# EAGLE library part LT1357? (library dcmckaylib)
High-speed (25MHz), high slew rate (600V/us) High bias current, 8nV/Hz^(0.5) voltage noise
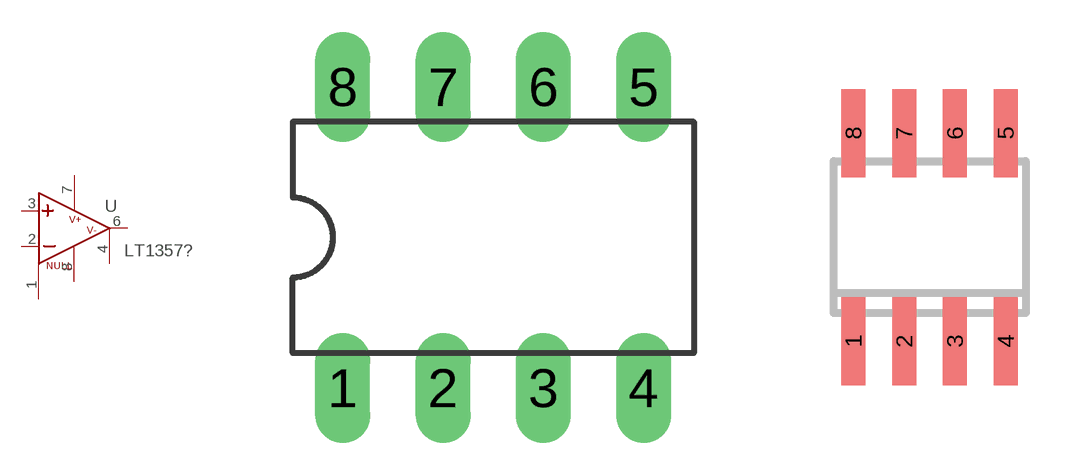
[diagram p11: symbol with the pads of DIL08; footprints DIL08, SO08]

Designator prefix U

## LT1357CN8  [DIL08]
1  NULL1
2  IN-  in
3  IN+  in
4  V-  pwr
6  OUT  out
7  V+  pwr
8  NULL2

## LT1357C38  [SO08]
Pads as for DIL08

## Footprint DIL08 (pad centres in mm)
Dual In Line Package
drill 0.889 long: 1 -3.81,-3.81; 2 -1.27,-3.81; 3 1.27,-3.81; 4 3.81,-3.81; 5 3.81,3.81; 6 1.27,3.81; 7 -1.27,3.81; 8 -3.81,3.81

## Footprint SO08 (pad centres in mm)
Small Outline Package 8 NS Package M08A
smd 0.6 x 2.2: 1 -1.905,-2.6; 2 -0.635,-2.6; 3 0.635,-2.6; 4 1.905,-2.6; 5 1.905,2.6; 6 0.635,2.6; 7 -0.635,2.6; 8 -1.905,2.6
